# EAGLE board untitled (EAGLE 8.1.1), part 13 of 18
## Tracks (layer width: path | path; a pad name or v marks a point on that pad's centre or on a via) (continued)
S$13047 (continued)
  Bottom 0: 298.18,114.21 298.3,114.24
S$13048
  Bottom 0: 298.3,114.24 297.54,113.48
S$13049
  Bottom 0: 297.54,113.48 297.49,113.43
S$13050
  Bottom 0: 297.49,113.43 297.45,113.37
S$13051
  Bottom 0: 297.45,113.37 297.42,113.3
S$13052
  Bottom 0: 297.42,113.3 297.41,113.24
S$13053
  Bottom 0: 297.41,113.24 297.4,113.17
S$13054
  Bottom 0: 297.4,113.17 297.4,112
S$13055
  Bottom 0: 297.4,112 296.57,111.17
S$13056
  Bottom 0: 248.77,112.57 248.77,125.97
S$13057
  Bottom 0: 248.77,125.97 248.84,126.02
S$13058
  Bottom 0: 248.84,126.02 248.97,126.23
S$13059
  Bottom 0: 248.97,126.23 249.02,126.48
S$13060
  Bottom 0: 249.02,126.48 248.97,126.73
S$13061
  Bottom 0: 248.97,126.73 248.84,126.94
S$13062
  Bottom 0: 248.84,126.94 248.77,127
S$13063
  Bottom 0: 248.77,127 248.77,135.59
S$13064
  Bottom 0: 248.77,135.59 257.07,143.89
S$13065
  Bottom 0: 257.07,143.89 257.07,143.68
S$13066
  Bottom 0: 257.07,143.68 257.15,143.37
S$13067
  Bottom 0: 257.15,143.37 257.32,143.09
S$13068
  Bottom 0: 257.32,143.09 257.56,142.87
S$13069
  Bottom 0: 257.56,142.87 257.85,142.72
S$13070
  Bottom 0: 257.85,142.72 258.17,142.66
S$13071
  Bottom 0: 258.17,142.66 258.5,142.68
S$13072
  Bottom 0: 258.5,142.68 258.71,142.75
S$13073
  Bottom 0: 258.71,142.75 259.77,141.7
S$13074
  Bottom 0: 259.77,141.7 259.73,141.68
S$13075
  Bottom 0: 259.73,141.68 259.67,141.62
S$13076
  Bottom 0: 259.67,141.62 259.63,141.55
S$13077
  Bottom 0: 259.63,141.55 259.62,141.48
S$13078
  Bottom 0: 259.62,141.48 259.62,139.7
S$13079
  Bottom 0: 259.62,139.7 259.63,139.62
S$13080
  Bottom 0: 259.63,139.62 259.67,139.55
S$13081
  Bottom 0: 259.67,139.55 259.73,139.5
S$13082
  Bottom 0: 259.73,139.5 259.8,139.46
S$13083
  Bottom 0: 259.8,139.46 259.87,139.45
S$13084
  Bottom 0: 259.87,139.45 261.36,139.45
S$13085
  Bottom 0: 261.36,139.45 257.23,135.32
S$13086
  Bottom 0: 257.23,135.32 257.17,135.25
S$13087
  Bottom 0: 257.17,135.25 257.12,135.18
S$13088
  Bottom 0: 257.12,135.18 257.09,135.1
S$13089
  Bottom 0: 257.09,135.1 257.07,135.01
S$13090
  Bottom 0: 257.07,135.01 257.06,134.92
S$13091
  Bottom 0: 257.06,134.92 257.06,122.61
S$13092
  Bottom 0: 257.06,122.61 257.04,122.63
S$13093
  Bottom 0: 257.04,122.63 256.97,122.67
S$13094
  Bottom 0: 256.97,122.67 256.89,122.68
S$13095
  Bottom 0: 256.89,122.68 255.11,122.68
S$13096
  Bottom 0: 255.11,122.68 255.04,122.67
S$13097
  Bottom 0: 255.04,122.67 254.97,122.63
S$13098
  Bottom 0: 254.97,122.63 254.91,122.58
S$13099
  Bottom 0: 254.91,122.58 254.87,122.5
S$13100
  Bottom 0: 254.87,122.5 254.86,122.43
S$13101
  Bottom 0: 254.86,122.43 254.86,120.65
S$13102
  Bottom 0: 254.86,120.65 254.87,120.57
S$13103
  Bottom 0: 254.87,120.57 254.91,120.5
S$13104
  Bottom 0: 254.91,120.5 254.97,120.45
S$13105
  Bottom 0: 254.97,120.45 255.04,120.41
S$13106
  Bottom 0: 255.04,120.41 255.11,120.4
S$13107
  Bottom 0: 255.11,120.4 256.6,120.4
S$13108
  Bottom 0: 256.6,120.4 248.77,112.57
S$13109
  Bottom 0: 302.63,114.76 302.56,114.85
S$13110
  Bottom 0: 302.56,114.85 302.3,115.08
S$13111
  Bottom 0: 302.3,115.08 301.98,115.23
S$13112
  Bottom 0: 301.98,115.23 301.63,115.29
S$13113
  Bottom 0: 301.63,115.29 301.29,115.27
S$13114
  Bottom 0: 301.29,115.27 301.18,115.23
S$13115
  Bottom 0: 301.18,115.23 300.87,115.29
S$13116
  Bottom 0: 300.87,115.29 300.58,115.28
S$13117
  Bottom 0: 300.58,115.28 300.6,115.3
S$13118
  Bottom 0: 300.6,115.3 300.65,115.35
S$13119
  Bottom 0: 300.65,115.35 300.69,115.41
S$13120
  Bottom 0: 300.69,115.41 300.72,115.47
S$13121
  Bottom 0: 300.72,115.47 300.73,115.54
S$13122
  Bottom 0: 300.73,115.54 300.74,115.61
S$13123
  Bottom 0: 300.74,115.61 300.74,123.98
S$13124
  Bottom 0: 300.74,123.98 300.9,123.81
S$13125
  Bottom 0: 300.9,123.81 301.03,123.75
S$13126
  Bottom 0: 301.03,123.75 301.03,121.64
S$13127
  Bottom 0: 301.03,121.64 301.03,121.54
S$13128
  Bottom 0: 301.03,121.54 301.05,121.46
S$13129
  Bottom 0: 301.05,121.46 301.09,121.38
S$13130
  Bottom 0: 301.09,121.38 301.13,121.3
S$13131
  Bottom 0: 301.13,121.3 301.19,121.23
S$13132
  Bottom 0: 301.19,121.23 302.63,119.8
S$13133
  Bottom 0: 302.63,119.8 302.63,114.76
S$13134
  Bottom 0: 109.4,115.7 109.49,116.01
S$13135
  Bottom 0: 109.49,116.01 109.54,116.46
S$13136
  Bottom 0: 109.54,116.46 109.49,116.91
S$13137
  Bottom 0: 109.49,116.91 109.37,117.33
S$13138
  Bottom 0: 109.37,117.33 109.15,117.73
S$13139
  Bottom 0: 109.15,117.73 108.87,118.07
S$13140
  Bottom 0: 108.87,118.07 108.52,118.36
S$13141
  Bottom 0: 108.52,118.36 108.13,118.57
S$13142
  Bottom 0: 108.13,118.57 107.7,118.7
S$13143
  Bottom 0: 107.7,118.7 107.25,118.75
S$13144
  Bottom 0: 107.25,118.75 106.81,118.7
S$13145
  Bottom 0: 106.81,118.7 106.38,118.57
S$13146
  Bottom 0: 106.38,118.57 105.98,118.36
S$13147
  Bottom 0: 105.98,118.36 105.64,118.07
S$13148
  Bottom 0: 105.64,118.07 105.35,117.73
S$13149
  Bottom 0: 105.35,117.73 105.14,117.33
S$13150
  Bottom 0: 105.14,117.33 105.01,116.91
S$13151
  Bottom 0: 105.01,116.91 104.97,116.46
S$13152
  Bottom 0: 104.97,116.46 105.01,116.01
S$13153
  Bottom 0: 105.01,116.01 105.1,115.72
S$13154
  Bottom 0: 105.1,115.72 96.31,124.5
S$13155
  Bottom 0: 96.31,124.5 103.58,131.77
S$13156
  Bottom 0: 103.58,131.77 103.64,131.84
S$13157
  Bottom 0: 103.64,131.84 103.68,131.91
S$13158
  Bottom 0: 103.68,131.91 103.72,131.99
S$13159
  Bottom 0: 103.72,131.99 103.74,132.08
S$13160
  Bottom 0: 103.74,132.08 103.74,132.17
S$13161
  Bottom 0: 103.74,132.17 103.74,141.64
S$13162
  Bottom 0: 103.74,141.64 114.43,141.64
S$13163
  Bottom 0: 114.43,141.64 114.41,141.62
S$13164
  Bottom 0: 114.41,141.62 114.37,141.55
S$13165
  Bottom 0: 114.37,141.55 114.36,141.48
S$13166
  Bottom 0: 114.36,141.48 114.36,139.7
S$13167
  Bottom 0: 114.36,139.7 114.37,139.62
S$13168
  Bottom 0: 114.37,139.62 114.41,139.55
S$13169
  Bottom 0: 114.41,139.55 114.47,139.5
S$13170
  Bottom 0: 114.47,139.5 114.54,139.46
S$13171
  Bottom 0: 114.54,139.46 114.61,139.45
S$13172
  Bottom 0: 114.61,139.45 116.39,139.45
S$13173
  Bottom 0: 116.39,139.45 116.47,139.46
S$13174
  Bottom 0: 116.47,139.46 116.54,139.5
S$13175
  Bottom 0: 116.54,139.5 116.6,139.55
S$13176
  Bottom 0: 116.6,139.55 116.64,139.62
S$13177
  Bottom 0: 116.64,139.62 116.65,139.7
S$13178
  Bottom 0: 116.65,139.7 116.65,141.48
S$13179
  Bottom 0: 116.65,141.48 116.64,141.55
S$13180
  Bottom 0: 116.64,141.55 116.6,141.62
S$13181
  Bottom 0: 116.6,141.62 116.58,141.64
S$13182
  Bottom 0: 116.58,141.64 117.61,141.64
S$13183
  Bottom 0: 117.61,141.64 117.57,141.63
S$13184
  Bottom 0: 117.57,141.63 117.3,141.45
S$13185
  Bottom 0: 117.3,141.45 117.08,141.21
S$13186
  Bottom 0: 117.08,141.21 116.94,140.91
S$13187
  Bottom 0: 116.94,140.91 116.9,140.59
S$13188
  Bottom 0: 116.9,140.59 116.94,140.27
S$13189
  Bottom 0: 116.94,140.27 117.08,139.97
S$13190
  Bottom 0: 117.08,139.97 117.3,139.72
S$13191
  Bottom 0: 117.3,139.72 117.57,139.55
S$13192
  Bottom 0: 117.57,139.55 117.88,139.46
S$13193
  Bottom 0: 117.88,139.46 118.21,139.46
S$13194
  Bottom 0: 118.21,139.46 118.52,139.55
S$13195
  Bottom 0: 118.52,139.55 118.79,139.72
S$13196
  Bottom 0: 118.79,139.72 119,139.97
S$13197
  Bottom 0: 119,139.97 119.14,140.27
S$13198
  Bottom 0: 119.14,140.27 119.19,140.59
S$13199
  Bottom 0: 119.19,140.59 119.14,140.91
S$13200
  Bottom 0: 119.14,140.91 119,141.21
S$13201
  Bottom 0: 119,141.21 118.79,141.45
S$13202
  Bottom 0: 118.79,141.45 118.52,141.63
S$13203
  Bottom 0: 118.52,141.63 118.48,141.64
S$13204
  Bottom 0: 118.48,141.64 118.96,141.64
S$13205
  Bottom 0: 118.96,141.64 119.04,141.65
S$13206
  Bottom 0: 119.04,141.65 119.14,141.67
S$13207
  Bottom 0: 119.14,141.67 119.22,141.7
S$13208
  Bottom 0: 119.22,141.7 119.29,141.75
S$13209
  Bottom 0: 119.29,141.75 119.36,141.81
S$13210
  Bottom 0: 119.36,141.81 120.26,142.71
S$13211
  Bottom 0: 120.26,142.71 120.52,142.66
S$13212
  Bottom 0: 120.52,142.66 120.84,142.68
S$13213
  Bottom 0: 120.84,142.68 121.15,142.78
S$13214
  Bottom 0: 121.15,142.78 121.41,142.97
S$13215
  Bottom 0: 121.41,142.97 121.51,143.09
S$13216
  Bottom 0: 121.51,143.09 121.51,137.35
S$13217
  Bottom 0: 121.51,137.35 118.92,134.76
S$13218
  Bottom 0: 118.92,134.76 119.01,135.06
S$13219
  Bottom 0: 119.01,135.06 119.06,135.51
S$13220
  Bottom 0: 119.06,135.51 119.01,135.96
S$13221
  Bottom 0: 119.01,135.96 118.89,136.38
S$13222
  Bottom 0: 118.89,136.38 118.67,136.78
S$13223
  Bottom 0: 118.67,136.78 118.39,137.12
S$13224
  Bottom 0: 118.39,137.12 118.04,137.41
S$13225
  Bottom 0: 118.04,137.41 117.64,137.62
S$13226
  Bottom 0: 117.64,137.62 117.22,137.75
S$13227
  Bottom 0: 117.22,137.75 116.77,137.79
S$13228
  Bottom 0: 116.77,137.79 116.33,137.75
S$13229
  Bottom 0: 116.33,137.75 115.9,137.62
S$13230
  Bottom 0: 115.9,137.62 115.5,137.41
S$13231
  Bottom 0: 115.5,137.41 115.16,137.12
S$13232
  Bottom 0: 115.16,137.12 114.87,136.78
S$13233
  Bottom 0: 114.87,136.78 114.66,136.38
S$13234
  Bottom 0: 114.66,136.38 114.53,135.96
S$13235
  Bottom 0: 114.53,135.96 114.49,135.51
S$13236
  Bottom 0: 114.49,135.51 114.53,135.06
S$13237
  Bottom 0: 114.53,135.06 114.66,134.63
S$13238
  Bottom 0: 114.66,134.63 114.87,134.24
S$13239
  Bottom 0: 114.87,134.24 115.16,133.89
S$13240
  Bottom 0: 115.16,133.89 115.5,133.61
S$13241
  Bottom 0: 115.5,133.61 115.9,133.4
S$13242
  Bottom 0: 115.9,133.4 116.33,133.27
S$13243
  Bottom 0: 116.33,133.27 116.77,133.22
S$13244
  Bottom 0: 116.77,133.22 117.22,133.27
S$13245
  Bottom 0: 117.22,133.27 117.52,133.35
S$13246
  Bottom 0: 117.52,133.35 116.34,132.18
S$13247
  Bottom 0: 116.34,132.18 116.29,132.12
S$13248
  Bottom 0: 116.29,132.12 116.25,132.06
S$13249
  Bottom 0: 116.25,132.06 116.22,132
S$13250
  Bottom 0: 116.22,132 116.21,131.93
S$13251
  Bottom 0: 116.21,131.93 116.2,131.86
S$13252
  Bottom 0: 116.2,131.86 116.2,130.76
S$13253
  Bottom 0: 116.2,130.76 115.59,130.15
S$13254
  Bottom 0: 115.59,130.15 115.63,130.43
S$13255
  Bottom 0: 115.63,130.43 115.58,130.77
S$13256
  Bottom 0: 115.58,130.77 115.46,131.1
S$13257
  Bottom 0: 115.46,131.1 115.25,131.38
S$13258
  Bottom 0: 115.25,131.38 114.98,131.61
S$13259
  Bottom 0: 114.98,131.61 114.67,131.76
S$13260
  Bottom 0: 114.67,131.76 114.32,131.82
S$13261
  Bottom 0: 114.32,131.82 113.97,131.8
S$13262
  Bottom 0: 113.97,131.8 113.64,131.69
S$13263
  Bottom 0: 113.64,131.69 113.61,131.68
S$13264
  Bottom 0: 113.61,131.68 113.04,132.25
S$13265
  Bottom 0: 113.04,132.25 112.99,132.29
S$13266
  Bottom 0: 112.99,132.29 112.93,132.33
S$13267
  Bottom 0: 112.93,132.33 112.87,132.35
S$13268
  Bottom 0: 112.87,132.35 112.8,132.37
S$13269
  Bottom 0: 112.8,132.37 112.73,132.38
S$13270
  Bottom 0: 112.73,132.38 108.16,132.38
S$13271
  Bottom 0: 108.16,132.38 108.1,132.51
S$13272
  Bottom 0: 108.1,132.51 107.89,132.72
S$13273
  Bottom 0: 107.89,132.72 107.63,132.88
S$13274
  Bottom 0: 107.63,132.88 107.33,132.94
S$13275
  Bottom 0: 107.33,132.94 107.03,132.92
S$13276
  Bottom 0: 107.03,132.92 106.75,132.81
S$13277
  Bottom 0: 106.75,132.81 106.51,132.62
S$13278
  Bottom 0: 106.51,132.62 106.34,132.38
S$13279
  Bottom 0: 106.34,132.38 106.25,132.09
S$13280
  Bottom 0: 106.25,132.09 106.25,131.78
S$13281
  Bottom 0: 106.25,131.78 106.34,131.49
S$13282
  Bottom 0: 106.34,131.49 106.51,131.24
S$13283
  Bottom 0: 106.51,131.24 106.75,131.05
S$13284
  Bottom 0: 106.75,131.05 107.03,130.94
S$13285
  Bottom 0: 107.03,130.94 107.33,130.92
S$13286
  Bottom 0: 107.33,130.92 107.63,130.99
S$13287
  Bottom 0: 107.63,130.99 107.89,131.14
S$13288
  Bottom 0: 107.89,131.14 108.1,131.36
S$13289
  Bottom 0: 108.1,131.36 108.16,131.49
S$13290
  Bottom 0: 108.16,131.49 112.54,131.49
S$13291
  Bottom 0: 112.54,131.49 112.99,131.04
S$13292
  Bottom 0: 112.99,131.04 112.93,130.94
S$13293
  Bottom 0: 112.93,130.94 112.85,130.6
S$13294
  Bottom 0: 112.85,130.6 112.85,130.25
S$13295
  Bottom 0: 112.85,130.25 112.93,129.92
S$13296
  Bottom 0: 112.93,129.92 113.1,129.61
S$13297
  Bottom 0: 113.1,129.61 113.34,129.35
S$13298
  Bottom 0: 113.34,129.35 113.64,129.16
S$13299
  Bottom 0: 113.64,129.16 113.97,129.06
S$13300
  Bottom 0: 113.97,129.06 114.32,129.04
S$13301
  Bottom 0: 114.32,129.04 114.52,129.07
S$13302
  Bottom 0: 114.52,129.07 112.12,126.67
S$13303
  Bottom 0: 112.12,126.67 110.5,126.67
S$13304
  Bottom 0: 110.5,126.67 110.43,126.67
S$13305
  Bottom 0: 110.43,126.67 110.37,126.66
S$13306
  Bottom 0: 110.37,126.66 110.31,126.63
S$13307
  Bottom 0: 110.31,126.63 110.25,126.59
S$13308
  Bottom 0: 110.25,126.59 110.19,126.55
S$13309
  Bottom 0: 110.19,126.55 106.92,123.28
S$13310
  Bottom 0: 106.92,123.28 106.88,123.23
S$13311
  Bottom 0: 106.88,123.23 106.84,123.17
S$13312
  Bottom 0: 106.84,123.17 106.82,123.1
S$13313
  Bottom 0: 106.82,123.1 106.8,123.04
S$13314
  Bottom 0: 106.8,123.04 106.8,122.97
S$13315
  Bottom 0: 106.8,122.97 106.8,122.68
S$13316
  Bottom 0: 106.8,122.68 106.43,122.68
S$13317
  Bottom 0: 106.43,122.68 106.43,122.81
S$13318
  Bottom 0: 106.43,122.81 106.36,123.03
S$13319
  Bottom 0: 106.36,123.03 106.2,123.19
S$13320
  Bottom 0: 106.2,123.19 105.98,123.25
S$13321
  Bottom 0: 105.98,123.25 105.63,123.25
S$13322
  Bottom 0: 105.63,123.25 104.54,124.34
S$13323
  Bottom 0: 104.54,124.34 104.6,124.47
S$13324
  Bottom 0: 104.6,124.47 104.65,124.8
S$13325
  Bottom 0: 104.65,124.8 104.6,125.11
S$13326
  Bottom 0: 104.6,125.11 104.47,125.42
S$13327
  Bottom 0: 104.47,125.42 104.27,125.67
S$13328
  Bottom 0: 104.27,125.67 104,125.86
S$13329
  Bottom 0: 104,125.86 103.7,125.96
S$13330
  Bottom 0: 103.7,125.96 103.37,125.98
S$13331
  Bottom 0: 103.37,125.98 103.05,125.92
S$13332
  Bottom 0: 103.05,125.92 102.76,125.77
S$13333
  Bottom 0: 102.76,125.77 102.53,125.55
S$13334
  Bottom 0: 102.53,125.55 102.36,125.27
S$13335
  Bottom 0: 102.36,125.27 102.27,124.96
S$13336
  Bottom 0: 102.27,124.96 102.27,124.63
S$13337
  Bottom 0: 102.27,124.63 102.36,124.32
S$13338
  Bottom 0: 102.36,124.32 102.53,124.04
S$13339
  Bottom 0: 102.53,124.04 102.76,123.82
S$13340
  Bottom 0: 102.76,123.82 103.05,123.67
S$13341
  Bottom 0: 103.05,123.67 103.37,123.61
S$13342
  Bottom 0: 103.37,123.61 103.7,123.63
S$13343
  Bottom 0: 103.7,123.63 103.92,123.7
S$13344
  Bottom 0: 103.92,123.7 104.97,122.65
S$13345
  Bottom 0: 104.97,122.65 104.94,122.63
S$13346
  Bottom 0: 104.94,122.63 104.89,122.58
S$13347
  Bottom 0: 104.89,122.58 104.85,122.5
S$13348
  Bottom 0: 104.85,122.5 104.84,122.43
S$13349
  Bottom 0: 104.84,122.43 104.84,120.65
S$13350
  Bottom 0: 104.84,120.65 104.85,120.57
S$13351
  Bottom 0: 104.85,120.57 104.89,120.5
S$13352
  Bottom 0: 104.89,120.5 104.94,120.45
S$13353
  Bottom 0: 104.94,120.45 105.02,120.41
S$13354
  Bottom 0: 105.02,120.41 105.09,120.4
S$13355
  Bottom 0: 105.09,120.4 106.61,120.4
S$13356
  Bottom 0: 106.61,120.4 104.36,118.15
S$13357
  Bottom 0: 104.36,118.15 104.12,118.12
S$13358
  Bottom 0: 104.12,118.12 103.9,118.01
S$13359
  Bottom 0: 103.9,118.01 103.73,117.83
S$13360
  Bottom 0: 103.73,117.83 103.64,117.59
S$13361
  Bottom 0: 103.64,117.59 103.64,117.34
S$13362
  Bottom 0: 103.64,117.34 103.73,117.1
S$13363
  Bottom 0: 103.73,117.1 103.9,116.92
S$13364
  Bottom 0: 103.9,116.92 104.12,116.8
S$13365
  Bottom 0: 104.12,116.8 104.37,116.78
S$13366
  Bottom 0: 104.37,116.78 104.62,116.85
S$13367
  Bottom 0: 104.62,116.85 104.82,117
S$13368
  Bottom 0: 104.82,117 104.95,117.22
S$13369
  Bottom 0: 104.95,117.22 105,117.47
S$13370
  Bottom 0: 105,117.47 104.99,117.51
S$13371
  Bottom 0: 104.99,117.51 107.55,120.08
S$13372
  Bottom 0: 107.55,120.08 107.59,120.13
S$13373
  Bottom 0: 107.59,120.13 107.64,120.19
S$13374
  Bottom 0: 107.64,120.19 107.66,120.25
S$13375
  Bottom 0: 107.66,120.25 107.67,120.32
S$13376
  Bottom 0: 107.67,120.32 107.68,120.39
S$13377
  Bottom 0: 107.68,120.39 107.68,120.79
S$13378
  Bottom 0: 107.68,120.79 107.78,120.67
S$13379
  Bottom 0: 107.78,120.67 108.05,120.5
S$13380
  Bottom 0: 108.05,120.5 108.36,120.41
S$13381
  Bottom 0: 108.36,120.41 108.69,120.41
S$13382
  Bottom 0: 108.69,120.41 109,120.5
S$13383
  Bottom 0: 109,120.5 109.27,120.67
S$13384
  Bottom 0: 109.27,120.67 109.48,120.92
S$13385
  Bottom 0: 109.48,120.92 109.62,121.22
S$13386
  Bottom 0: 109.62,121.22 109.67,121.54
S$13387
  Bottom 0: 109.67,121.54 109.62,121.86
S$13388
  Bottom 0: 109.62,121.86 109.48,122.16
S$13389
  Bottom 0: 109.48,122.16 109.27,122.4
S$13390
  Bottom 0: 109.27,122.4 109,122.58
S$13391
  Bottom 0: 109,122.58 108.69,122.67
S$13392
  Bottom 0: 108.69,122.67 108.36,122.67
S$13393
  Bottom 0: 108.36,122.67 108.05,122.58
S$13394
  Bottom 0: 108.05,122.58 107.78,122.4
S$13395
  Bottom 0: 107.78,122.4 107.68,122.29
S$13396
  Bottom 0: 107.68,122.29 107.68,122.78
S$13397
  Bottom 0: 107.68,122.78 109.9,125
S$13398
  Bottom 0: 109.9,125 109.89,124.96
S$13399
  Bottom 0: 109.89,124.96 109.89,124.63
S$13400
  Bottom 0: 109.89,124.63 109.98,124.32
S$13401
  Bottom 0: 109.98,124.32 110.15,124.04
S$13402
  Bottom 0: 110.15,124.04 110.38,123.82
S$13403
  Bottom 0: 110.38,123.82 110.5,123.76
S$13404
  Bottom 0: 110.5,123.76 110.5,116.8
S$13405
  Bottom 0: 110.5,116.8 109.4,115.7
S$13406
  Bottom 0: 107.33,138.54 107.63,138.61
S$13407
  Bottom 0: 107.63,138.61 107.89,138.76
S$13408
  Bottom 0: 107.89,138.76 108.1,138.98
S$13409
  Bottom 0: 108.1,138.98 108.23,139.25
S$13410
  Bottom 0: 108.23,139.25 108.28,139.55
S$13411
  Bottom 0: 108.28,139.55 108.23,139.85
S$13412
  Bottom 0: 108.23,139.85 108.1,140.13
S$13413
  Bottom 0: 108.1,140.13 107.89,140.34
S$13414
  Bottom 0: 107.89,140.34 107.63,140.5
S$13415
  Bottom 0: 107.63,140.5 107.33,140.56
S$13416
  Bottom 0: 107.33,140.56 107.03,140.54
S$13417
  Bottom 0: 107.03,140.54 106.75,140.43
S$13418
  Bottom 0: 106.75,140.43 106.51,140.24
S$13419
  Bottom 0: 106.51,140.24 106.34,140
S$13420
  Bottom 0: 106.34,140 106.25,139.71
S$13421
  Bottom 0: 106.25,139.71 106.25,139.4
S$13422
  Bottom 0: 106.25,139.4 106.34,139.11
S$13423
  Bottom 0: 106.34,139.11 106.51,138.86
S$13424
  Bottom 0: 106.51,138.86 106.75,138.67
S$13425
  Bottom 0: 106.75,138.67 107.03,138.56
S$13426
  Bottom 0: 107.03,138.56 107.33,138.54
S$13427
  Bottom 0: 147.56,117.01 147.46,117.33
S$13428
  Bottom 0: 147.46,117.33 147.25,117.73
S$13429
  Bottom 0: 147.25,117.73 146.96,118.07
S$13430
  Bottom 0: 146.96,118.07 146.62,118.36
S$13431
  Bottom 0: 146.62,118.36 146.22,118.57
S$13432
  Bottom 0: 146.22,118.57 145.8,118.7
S$13433
  Bottom 0: 145.8,118.7 145.35,118.75
S$13434
  Bottom 0: 145.35,118.75 144.9,118.7
S$13435
  Bottom 0: 144.9,118.7 144.47,118.57
S$13436
  Bottom 0: 144.47,118.57 144.42,118.55
S$13437
  Bottom 0: 144.42,118.55 146.32,120.45
S$13438
  Bottom 0: 146.32,120.45 146.46,120.41
S$13439
  Bottom 0: 146.46,120.41 146.78,120.41
S$13440
  Bottom 0: 146.78,120.41 147.09,120.5
S$13441
  Bottom 0: 147.09,120.5 147.36,120.67
S$13442
  Bottom 0: 147.36,120.67 147.56,120.89
S$13443
  Bottom 0: 147.56,120.89 147.56,117.01
S$13444
  Bottom 0: 142.11,117.84 137.75,122.2
S$13445
  Bottom 0: 137.75,122.2 137.69,122.26
S$13446
  Bottom 0: 137.69,122.26 137.61,122.31
S$13447
  Bottom 0: 137.61,122.31 137.53,122.34
S$13448
  Bottom 0: 137.53,122.34 137.44,122.36
S$13449
  Bottom 0: 137.44,122.36 137.35,122.37
S$13450
  Bottom 0: 137.35,122.37 128.34,122.37
S$13451
  Bottom 0: 128.34,122.37 128.31,122.4
S$13452
  Bottom 0: 128.31,122.4 128.04,122.58
S$13453
  Bottom 0: 128.04,122.58 127.73,122.67
S$13454
  Bottom 0: 127.73,122.67 127.41,122.67
S$13455
  Bottom 0: 127.41,122.67 127.1,122.58
S$13456
  Bottom 0: 127.1,122.58 126.82,122.4
S$13457
  Bottom 0: 126.82,122.4 126.61,122.16
S$13458
  Bottom 0: 126.61,122.16 126.47,121.86
S$13459
  Bottom 0: 126.47,121.86 126.43,121.54
S$13460
  Bottom 0: 126.43,121.54 126.47,121.22
S$13461
  Bottom 0: 126.47,121.22 126.61,120.92
S$13462
  Bottom 0: 126.61,120.92 126.82,120.67
S$13463
  Bottom 0: 126.82,120.67 127,120.56
S$13464
  Bottom 0: 127,120.56 126.15,120.56
S$13465
  Bottom 0: 126.15,120.56 126.16,120.57
S$13466
  Bottom 0: 126.16,120.57 126.17,120.65
S$13467
  Bottom 0: 126.17,120.65 126.17,122.43
S$13468
  Bottom 0: 126.17,122.43 126.16,122.5
S$13469
  Bottom 0: 126.16,122.5 126.12,122.58
S$13470
  Bottom 0: 126.12,122.58 126.06,122.63
S$13471
  Bottom 0: 126.06,122.63 125.99,122.67
S$13472
  Bottom 0: 125.99,122.67 125.92,122.68
S$13473
  Bottom 0: 125.92,122.68 125.47,122.68
S$13474
  Bottom 0: 125.47,122.68 125.47,122.81
S$13475
  Bottom 0: 125.47,122.81 125.41,123.03
S$13476
  Bottom 0: 125.41,123.03 125.25,123.19
S$13477
  Bottom 0: 125.25,123.19 125.03,123.25
S$13478
  Bottom 0: 125.03,123.25 124.68,123.25
S$13479
  Bottom 0: 124.68,123.25 123.59,124.34
S$13480
  Bottom 0: 123.59,124.34 123.65,124.47
S$13481
  Bottom 0: 123.65,124.47 123.7,124.8
S$13482
  Bottom 0: 123.7,124.8 123.65,125.11
S$13483
  Bottom 0: 123.65,125.11 123.53,125.42
S$13484
  Bottom 0: 123.53,125.42 123.32,125.67
S$13485
  Bottom 0: 123.32,125.67 123.05,125.86
S$13486
  Bottom 0: 123.05,125.86 122.75,125.96
S$13487
  Bottom 0: 122.75,125.96 122.42,125.98
S$13488
  Bottom 0: 122.42,125.98 122.1,125.92
S$13489
  Bottom 0: 122.1,125.92 121.81,125.77
S$13490
  Bottom 0: 121.81,125.77 121.58,125.55
S$13491
  Bottom 0: 121.58,125.55 121.41,125.27
S$13492
  Bottom 0: 121.41,125.27 121.32,124.96
S$13493
  Bottom 0: 121.32,124.96 121.32,124.63
S$13494
  Bottom 0: 121.32,124.63 121.41,124.32
S$13495
  Bottom 0: 121.41,124.32 121.58,124.04
S$13496
  Bottom 0: 121.58,124.04 121.81,123.82
S$13497
  Bottom 0: 121.81,123.82 122.1,123.67
S$13498
  Bottom 0: 122.1,123.67 122.42,123.61
S$13499
  Bottom 0: 122.42,123.61 122.75,123.63
S$13500
  Bottom 0: 122.75,123.63 122.97,123.7
S$13501
  Bottom 0: 122.97,123.7 124.02,122.65
S$13502
  Bottom 0: 124.02,122.65 123.99,122.63
S$13503
  Bottom 0: 123.99,122.63 123.94,122.58
S$13504
  Bottom 0: 123.94,122.58 123.9,122.5
S$13505
  Bottom 0: 123.9,122.5 123.89,122.43
S$13506
  Bottom 0: 123.89,122.43 123.89,120.65
S$13507
  Bottom 0: 123.89,120.65 123.9,120.57
S$13508
  Bottom 0: 123.9,120.57 123.91,120.56
S$13509
  Bottom 0: 123.91,120.56 117.79,120.56
S$13510
  Bottom 0: 117.79,120.56 117.75,120.8
S$13511
  Bottom 0: 117.75,120.8 117.62,121.08
S$13512
  Bottom 0: 117.62,121.08 117.42,121.3
S$13513
  Bottom 0: 117.42,121.3 117.16,121.45
S$13514
  Bottom 0: 117.16,121.45 116.86,121.51
S$13515
  Bottom 0: 116.86,121.51 116.81,121.51
S$13516
  Bottom 0: 116.81,121.51 123.67,128.37
S$13517
  Bottom 0: 123.67,128.37 137.68,128.37
S$13518
  Bottom 0: 137.68,128.37 137.75,128.38
S$13519
  Bottom 0: 137.75,128.38 137.81,128.39
S$13520
  Bottom 0: 137.81,128.39 137.88,128.42
S$13521
  Bottom 0: 137.88,128.42 137.94,128.46
S$13522
  Bottom 0: 137.94,128.46 137.99,128.5
S$13523
  Bottom 0: 137.99,128.5 149.31,139.82
S$13524
  Bottom 0: 149.31,139.82 149.33,139.84
S$13525
  Bottom 0: 149.33,139.84 149.33,138.24
S$13526
  Bottom 0: 149.33,138.24 143.87,132.78
S$13527
  Bottom 0: 143.87,132.78 143.82,132.72
S$13528
  Bottom 0: 143.82,132.72 143.78,132.66
S$13529
  Bottom 0: 143.78,132.66 143.76,132.6
S$13530
  Bottom 0: 143.76,132.6 143.74,132.53
S$13531
  Bottom 0: 143.74,132.53 143.74,132.46
S$13532
  Bottom 0: 143.74,132.46 143.74,128.37
S$13533
  Bottom 0: 143.74,128.37 143.74,128.3
S$13534
  Bottom 0: 143.74,128.3 143.76,128.23
S$13535
  Bottom 0: 143.76,128.23 143.78,128.17
S$13536
  Bottom 0: 143.78,128.17 143.82,128.11
S$13537
  Bottom 0: 143.82,128.11 143.87,128.06
S$13538
  Bottom 0: 143.87,128.06 144.96,126.96
S$13539
  Bottom 0: 144.96,126.96 144.96,126.79
S$13540
  Bottom 0: 144.96,126.79 145.05,126.55
S$13541
  Bottom 0: 145.05,126.55 145.22,126.36
S$13542
  Bottom 0: 145.22,126.36 145.44,126.25
S$13543
  Bottom 0: 145.44,126.25 145.69,126.23
S$13544
  Bottom 0: 145.69,126.23 145.94,126.3
S$13545
  Bottom 0: 145.94,126.3 146.05,126.38
S$13546
  Bottom 0: 146.05,126.38 146.05,122.52
S$13547
  Bottom 0: 146.05,122.52 145.87,122.4
S$13548
  Bottom 0: 145.87,122.4 145.66,122.16
S$13549
  Bottom 0: 145.66,122.16 145.52,121.86
S$13550
  Bottom 0: 145.52,121.86 145.48,121.54
S$13551
  Bottom 0: 145.48,121.54 145.52,121.24
S$13552
  Bottom 0: 145.52,121.24 145.22,120.94
S$13553
  Bottom 0: 145.22,120.94 145.22,122.43
S$13554
  Bottom 0: 145.22,122.43 145.21,122.5
S$13555
  Bottom 0: 145.21,122.5 145.17,122.58
S$13556
  Bottom 0: 145.17,122.58 145.12,122.63
S$13557
  Bottom 0: 145.12,122.63 145.04,122.67
S$13558
  Bottom 0: 145.04,122.67 144.97,122.68
S$13559
  Bottom 0: 144.97,122.68 144.52,122.68
S$13560
  Bottom 0: 144.52,122.68 144.52,122.81
S$13561
  Bottom 0: 144.52,122.81 144.46,123.03
S$13562
  Bottom 0: 144.46,123.03 144.3,123.19
S$13563
  Bottom 0: 144.3,123.19 144.08,123.25
S$13564
  Bottom 0: 144.08,123.25 143.72,123.25
S$13565
  Bottom 0: 143.72,123.25 142.64,124.33
S$13566
  Bottom 0: 142.64,124.33 142.7,124.47
S$13567
  Bottom 0: 142.7,124.47 142.75,124.79
S$13568
  Bottom 0: 142.75,124.79 142.7,125.11
S$13569
  Bottom 0: 142.7,125.11 142.57,125.41
S$13570
  Bottom 0: 142.57,125.41 142.37,125.66
S$13571
  Bottom 0: 142.37,125.66 142.1,125.85
S$13572
  Bottom 0: 142.1,125.85 141.8,125.96
S$13573
  Bottom 0: 141.8,125.96 141.47,125.98
S$13574
  Bottom 0: 141.47,125.98 141.15,125.91
S$13575
  Bottom 0: 141.15,125.91 140.86,125.77
S$13576
  Bottom 0: 140.86,125.77 140.63,125.54
S$13577
  Bottom 0: 140.63,125.54 140.46,125.27
S$13578
  Bottom 0: 140.46,125.27 140.37,124.95
S$13579
  Bottom 0: 140.37,124.95 140.37,124.63
S$13580
  Bottom 0: 140.37,124.63 140.46,124.31
S$13581
  Bottom 0: 140.46,124.31 140.63,124.04
S$13582
  Bottom 0: 140.63,124.04 140.86,123.81
S$13583
  Bottom 0: 140.86,123.81 141.15,123.67
S$13584
  Bottom 0: 141.15,123.67 141.47,123.6
S$13585
  Bottom 0: 141.47,123.6 141.8,123.62
S$13586
  Bottom 0: 141.8,123.62 142.02,123.7
S$13587
  Bottom 0: 142.02,123.7 143.07,122.65
S$13588
  Bottom 0: 143.07,122.65 143.04,122.63
S$13589
  Bottom 0: 143.04,122.63 142.99,122.58
S$13590
  Bottom 0: 142.99,122.58 142.95,122.5
S$13591
  Bottom 0: 142.95,122.5 142.94,122.43
S$13592
  Bottom 0: 142.94,122.43 142.94,120.65
S$13593
  Bottom 0: 142.94,120.65 142.95,120.57
S$13594
  Bottom 0: 142.95,120.57 142.99,120.5
S$13595
  Bottom 0: 142.99,120.5 143.04,120.45
S$13596
  Bottom 0: 143.04,120.45 143.11,120.41
S$13597
  Bottom 0: 143.11,120.41 143.19,120.4
S$13598
  Bottom 0: 143.19,120.4 144.67,120.4
S$13599
  Bottom 0: 144.67,120.4 142.11,117.84
S$13600
  Bottom 0: 130.04,123.61 130.37,123.63
S$13601
  Bottom 0: 130.37,123.63 130.67,123.73
S$13602
  Bottom 0: 130.67,123.73 130.94,123.92
S$13603
  Bottom 0: 130.94,123.92 131.15,124.18
S$13604
  Bottom 0: 131.15,124.18 131.27,124.47
S$13605
  Bottom 0: 131.27,124.47 131.32,124.8
S$13606
  Bottom 0: 131.32,124.8 131.27,125.11
S$13607
  Bottom 0: 131.27,125.11 131.15,125.42
S$13608
  Bottom 0: 131.15,125.42 130.94,125.67
S$13609
  Bottom 0: 130.94,125.67 130.67,125.86
S$13610
  Bottom 0: 130.67,125.86 130.37,125.96
S$13611
  Bottom 0: 130.37,125.96 130.04,125.98
S$13612
  Bottom 0: 130.04,125.98 129.72,125.92
S$13613
  Bottom 0: 129.72,125.92 129.43,125.77
S$13614
  Bottom 0: 129.43,125.77 129.2,125.55
S$13615
  Bottom 0: 129.2,125.55 129.03,125.27
S$13616
  Bottom 0: 129.03,125.27 128.94,124.96
S$13617
  Bottom 0: 128.94,124.96 128.94,124.63
S$13618
  Bottom 0: 128.94,124.63 129.03,124.32
S$13619
  Bottom 0: 129.03,124.32 129.2,124.04
S$13620
  Bottom 0: 129.2,124.04 129.43,123.82
S$13621
  Bottom 0: 129.43,123.82 129.72,123.67
S$13622
  Bottom 0: 129.72,123.67 130.04,123.61
S$13623
  Bottom 0: 90.08,120.59 90.21,120.67
S$13624
  Bottom 0: 90.21,120.67 90.43,120.92
S$13625
  Bottom 0: 90.43,120.92 90.56,121.22
S$13626
  Bottom 0: 90.56,121.22 90.61,121.54
S$13627
  Bottom 0: 90.61,121.54 90.56,121.86
S$13628
  Bottom 0: 90.56,121.86 90.43,122.16
S$13629
  Bottom 0: 90.43,122.16 90.21,122.4
S$13630
  Bottom 0: 90.21,122.4 90.04,122.52
S$13631
  Bottom 0: 90.04,122.52 90.04,131.01
S$13632
  Bottom 0: 90.04,131.01 91.23,132.2
S$13633
  Bottom 0: 91.23,132.2 91.26,132.2
S$13634
  Bottom 0: 91.26,132.2 91.34,132.22
S$13635
  Bottom 0: 91.34,132.22 91.42,132.25
S$13636
  Bottom 0: 91.42,132.25 91.5,132.3
S$13637
  Bottom 0: 91.5,132.3 91.57,132.36
S$13638
  Bottom 0: 91.57,132.36 95.64,136.43
S$13639
  Bottom 0: 95.64,136.43 95.61,136.38
S$13640
  Bottom 0: 95.61,136.38 95.48,135.96
S$13641
  Bottom 0: 95.48,135.96 95.44,135.51
S$13642
  Bottom 0: 95.44,135.51 95.48,135.06
S$13643
  Bottom 0: 95.48,135.06 95.61,134.63
S$13644
  Bottom 0: 95.61,134.63 95.82,134.24
S$13645
  Bottom 0: 95.82,134.24 96.11,133.89
S$13646
  Bottom 0: 96.11,133.89 96.45,133.61
S$13647
  Bottom 0: 96.45,133.61 96.85,133.4
S$13648
  Bottom 0: 96.85,133.4 97.28,133.27
S$13649
  Bottom 0: 97.28,133.27 97.72,133.22
S$13650
  Bottom 0: 97.72,133.22 98.17,133.27
S$13651
  Bottom 0: 98.17,133.27 98.59,133.4
S$13652
  Bottom 0: 98.59,133.4 98.99,133.61
S$13653
  Bottom 0: 98.99,133.61 99.34,133.89
S$13654
  Bottom 0: 99.34,133.89 99.62,134.24
S$13655
  Bottom 0: 99.62,134.24 99.83,134.63
S$13656
  Bottom 0: 99.83,134.63 99.96,135.06
S$13657
  Bottom 0: 99.96,135.06 100.01,135.51
S$13658
  Bottom 0: 100.01,135.51 99.96,135.96
S$13659
  Bottom 0: 99.96,135.96 99.83,136.38
S$13660
  Bottom 0: 99.83,136.38 99.62,136.78
S$13661
  Bottom 0: 99.62,136.78 99.34,137.12
S$13662
  Bottom 0: 99.34,137.12 98.99,137.41
S$13663
  Bottom 0: 98.99,137.41 98.59,137.62
S$13664
  Bottom 0: 98.59,137.62 98.17,137.75
S$13665
  Bottom 0: 98.17,137.75 97.72,137.79
S$13666
  Bottom 0: 97.72,137.79 97.28,137.75
S$13667
  Bottom 0: 97.28,137.75 96.85,137.62
S$13668
  Bottom 0: 96.85,137.62 96.8,137.6
S$13669
  Bottom 0: 96.8,137.6 98.7,139.5
S$13670
  Bottom 0: 98.7,139.5 98.83,139.46
S$13671
  Bottom 0: 98.83,139.46 99.16,139.46
S$13672
  Bottom 0: 99.16,139.46 99.47,139.55
S$13673
  Bottom 0: 99.47,139.55 99.74,139.72
S$13674
  Bottom 0: 99.74,139.72 99.95,139.97
S$13675
  Bottom 0: 99.95,139.97 100.09,140.27
S$13676
  Bottom 0: 100.09,140.27 100.14,140.59
S$13677
  Bottom 0: 100.14,140.59 100.14,140.61
S$13678
  Bottom 0: 100.14,140.61 101.09,139.65
S$13679
  Bottom 0: 101.09,139.65 101.09,134.28
S$13680
  Bottom 0: 101.09,134.28 100.94,134.23
S$13681
  Bottom 0: 100.94,134.23 100.64,134.05
S$13682
  Bottom 0: 100.64,134.05 100.4,133.79
S$13683
  Bottom 0: 100.4,133.79 100.23,133.48
S$13684
  Bottom 0: 100.23,133.48 100.15,133.14
S$13685
  Bottom 0: 100.15,133.14 100.15,132.79
S$13686
  Bottom 0: 100.15,132.79 100.23,132.46
S$13687
  Bottom 0: 100.23,132.46 100.4,132.15
S$13688
  Bottom 0: 100.4,132.15 100.64,131.89
S$13689
  Bottom 0: 100.64,131.89 100.94,131.7
S$13690
  Bottom 0: 100.94,131.7 101.27,131.6
S$13691
  Bottom 0: 101.27,131.6 101.62,131.58
S$13692
  Bottom 0: 101.62,131.58 101.81,131.61
S$13693
  Bottom 0: 101.81,131.61 95.49,125.29
S$13694
  Bottom 0: 95.49,125.29 95.48,125.3
S$13695
  Bottom 0: 95.48,125.3 95.4,125.33
S$13696
  Bottom 0: 95.4,125.33 95.31,125.35
S$13697
  Bottom 0: 95.31,125.35 95.22,125.36
S$13698
  Bottom 0: 95.22,125.36 93.06,125.36
S$13699
  Bottom 0: 93.06,125.36 93.04,125.41
S$13700
  Bottom 0: 93.04,125.41 92.83,125.66
S$13701
  Bottom 0: 92.83,125.66 92.57,125.85
S$13702
  Bottom 0: 92.57,125.85 92.26,125.96
S$13703
  Bottom 0: 92.26,125.96 91.94,125.98
S$13704
  Bottom 0: 91.94,125.98 91.62,125.91
S$13705
  Bottom 0: 91.62,125.91 91.33,125.77
S$13706
  Bottom 0: 91.33,125.77 91.09,125.54
S$13707
  Bottom 0: 91.09,125.54 90.92,125.27
S$13708
  Bottom 0: 90.92,125.27 90.83,124.95
S$13709
  Bottom 0: 90.83,124.95 90.83,124.63
S$13710
  Bottom 0: 90.83,124.63 90.92,124.31
S$13711
  Bottom 0: 90.92,124.31 91.09,124.04
S$13712
  Bottom 0: 91.09,124.04 91.33,123.81
S$13713
  Bottom 0: 91.33,123.81 91.62,123.67
S$13714
  Bottom 0: 91.62,123.67 91.94,123.6
S$13715
  Bottom 0: 91.94,123.6 92.26,123.62
S$13716
  Bottom 0: 92.26,123.62 92.57,123.73
S$13717
  Bottom 0: 92.57,123.73 92.83,123.92
S$13718
  Bottom 0: 92.83,123.92 93.04,124.17
S$13719
  Bottom 0: 93.04,124.17 93.06,124.22
S$13720
  Bottom 0: 93.06,124.22 94.99,124.22
S$13721
  Bottom 0: 94.99,124.22 95.11,124.1
S$13722
  Bottom 0: 95.11,124.1 97.7,121.51
S$13723
  Bottom 0: 97.7,121.51 97.51,121.49
S$13724
  Bottom 0: 97.51,121.49 97.23,121.38
S$13725
  Bottom 0: 97.23,121.38 96.99,121.19
S$13726
  Bottom 0: 96.99,121.19 96.82,120.94
S$13727
  Bottom 0: 96.82,120.94 96.73,120.66
S$13728
  Bottom 0: 96.73,120.66 96.73,120.59
S$13729
  Bottom 0: 96.73,120.59 90.08,120.59
S$13730
  Bottom 0: 95.27,129.04 95.62,129.1
S$13731
  Bottom 0: 95.62,129.1 95.93,129.25
S$13732
  Bottom 0: 95.93,129.25 96.2,129.47
S$13733
  Bottom 0: 96.2,129.47 96.41,129.76
S$13734
  Bottom 0: 96.41,129.76 96.53,130.08
S$13735
  Bottom 0: 96.53,130.08 96.58,130.43
S$13736
  Bottom 0: 96.58,130.43 96.53,130.77
S$13737
  Bottom 0: 96.53,130.77 96.41,131.1
S$13738
  Bottom 0: 96.41,131.1 96.2,131.38
S$13739
  Bottom 0: 96.2,131.38 95.93,131.61
S$13740
  Bottom 0: 95.93,131.61 95.62,131.76
S$13741
  Bottom 0: 95.62,131.76 95.27,131.82
S$13742
  Bottom 0: 95.27,131.82 94.92,131.8
S$13743
  Bottom 0: 94.92,131.8 94.59,131.69
S$13744
  Bottom 0: 94.59,131.69 94.3,131.51
S$13745
  Bottom 0: 94.3,131.51 94.05,131.25
S$13746
  Bottom 0: 94.05,131.25 93.88,130.94
S$13747
  Bottom 0: 93.88,130.94 93.8,130.6
S$13748
  Bottom 0: 93.8,130.6 93.8,130.25
S$13749
  Bottom 0: 93.8,130.25 93.88,129.92
S$13750
  Bottom 0: 93.88,129.92 94.05,129.61
S$13751
  Bottom 0: 94.05,129.61 94.3,129.35
S$13752
  Bottom 0: 94.3,129.35 94.59,129.16
S$13753
  Bottom 0: 94.59,129.16 94.92,129.06
S$13754
  Bottom 0: 94.92,129.06 95.27,129.04
S$13755
  Bottom 0: 185.7,122.11 185.68,122.16
S$13756
  Bottom 0: 185.68,122.16 185.47,122.4
S$13757
  Bottom 0: 185.47,122.4 185.19,122.58
S$13758
  Bottom 0: 185.19,122.58 185.16,122.59
S$13759
  Bottom 0: 185.16,122.59 185.64,122.59
S$13760
  Bottom 0: 185.64,122.59 185.72,122.6
S$13761
  Bottom 0: 185.72,122.6 185.82,122.62
S$13762
  Bottom 0: 185.82,122.62 185.9,122.65
S$13763
  Bottom 0: 185.9,122.65 185.97,122.7
S$13764
  Bottom 0: 185.97,122.7 186.04,122.76
S$13765
  Bottom 0: 186.04,122.76 186.94,123.66
S$13766
  Bottom 0: 186.94,123.66 187.2,123.61
S$13767
  Bottom 0: 187.2,123.61 187.52,123.63
S$13768
  Bottom 0: 187.52,123.63 187.83,123.73
S$13769
  Bottom 0: 187.83,123.73 188.09,123.92
S$13770
  Bottom 0: 188.09,123.92 188.3,124.18
S$13771
  Bottom 0: 188.3,124.18 188.43,124.47
S$13772
  Bottom 0: 188.43,124.47 188.47,124.8
S$13773
  Bottom 0: 188.47,124.8 188.43,125.11
S$13774
  Bottom 0: 188.43,125.11 188.3,125.42
S$13775
  Bottom 0: 188.3,125.42 188.09,125.67
S$13776
  Bottom 0: 188.09,125.67 187.83,125.86
S$13777
  Bottom 0: 187.83,125.86 187.52,125.96
S$13778
  Bottom 0: 187.52,125.96 187.2,125.98
S$13779
  Bottom 0: 187.2,125.98 186.88,125.92
S$13780
  Bottom 0: 186.88,125.92 186.59,125.77
S$13781
  Bottom 0: 186.59,125.77 186.35,125.55
S$13782
  Bottom 0: 186.35,125.55 186.18,125.27
S$13783
  Bottom 0: 186.18,125.27 186.1,124.96
S$13784
  Bottom 0: 186.1,124.96 186.1,124.63
S$13785
  Bottom 0: 186.1,124.63 186.14,124.47
S$13786
  Bottom 0: 186.14,124.47 185.41,123.73
S$13787
  Bottom 0: 185.41,123.73 180.19,123.73
S$13788
  Bottom 0: 180.19,123.73 180.21,123.73
S$13789
  Bottom 0: 180.21,123.73 180.47,123.92
S$13790
  Bottom 0: 180.47,123.92 180.68,124.18
S$13791
  Bottom 0: 180.68,124.18 180.81,124.47
S$13792
  Bottom 0: 180.81,124.47 180.85,124.8
S$13793
  Bottom 0: 180.85,124.8 180.81,125.11
S$13794
  Bottom 0: 180.81,125.11 180.68,125.42
S$13795
  Bottom 0: 180.68,125.42 180.47,125.67
S$13796
  Bottom 0: 180.47,125.67 180.21,125.86
S$13797
  Bottom 0: 180.21,125.86 179.9,125.96
S$13798
  Bottom 0: 179.9,125.96 179.58,125.98
S$13799
  Bottom 0: 179.58,125.98 179.26,125.92
S$13800
  Bottom 0: 179.26,125.92 178.97,125.77
S$13801
  Bottom 0: 178.97,125.77 178.74,125.55
S$13802
  Bottom 0: 178.74,125.55 178.66,125.42
S$13803
  Bottom 0: 178.66,125.42 178.66,126.22
S$13804
  Bottom 0: 178.66,126.22 179.79,127.35
S$13805
  Bottom 0: 179.79,127.35 179.85,127.42
S$13806
  Bottom 0: 179.85,127.42 179.9,127.49
S$13807
  Bottom 0: 179.9,127.49 179.93,127.57
S$13808
  Bottom 0: 179.93,127.57 179.95,127.66
S$13809
  Bottom 0: 179.95,127.66 179.96,127.75
S$13810
  Bottom 0: 179.96,127.75 179.96,141.64
S$13811
  Bottom 0: 179.96,141.64 188.25,141.64
S$13812
  Bottom 0: 188.25,141.64 188.2,141.58
S$13813
  Bottom 0: 188.2,141.58 188.11,141.35
S$13814
  Bottom 0: 188.11,141.35 188.11,141.09
S$13815
  Bottom 0: 188.11,141.09 188.2,140.86
S$13816
  Bottom 0: 188.2,140.86 188.37,140.67
S$13817
  Bottom 0: 188.37,140.67 188.59,140.56
S$13818
  Bottom 0: 188.59,140.56 190.8,138.35
S$13819
  Bottom 0: 190.8,138.35 190.85,138.31
S$13820
  Bottom 0: 190.85,138.31 190.91,138.27
S$13821
  Bottom 0: 190.91,138.27 190.97,138.25
S$13822
  Bottom 0: 190.97,138.25 191.04,138.23
S$13823
  Bottom 0: 191.04,138.23 191.11,138.23
S$13824
  Bottom 0: 191.11,138.23 193.03,138.23
S$13825
  Bottom 0: 193.03,138.23 193.54,137.71
S$13826
  Bottom 0: 193.54,137.71 193.42,137.75
S$13827
  Bottom 0: 193.42,137.75 192.97,137.79
S$13828
  Bottom 0: 192.97,137.79 192.53,137.75
S$13829
  Bottom 0: 192.53,137.75 192.1,137.62
S$13830
  Bottom 0: 192.1,137.62 191.7,137.41
S$13831
  Bottom 0: 191.7,137.41 191.36,137.12
S$13832
  Bottom 0: 191.36,137.12 191.07,136.78
S$13833
  Bottom 0: 191.07,136.78 190.86,136.38
S$13834
  Bottom 0: 190.86,136.38 190.73,135.96
S$13835
  Bottom 0: 190.73,135.96 190.69,135.51
S$13836
  Bottom 0: 190.69,135.51 190.73,135.06
S$13837
  Bottom 0: 190.73,135.06 190.86,134.63
S$13838
  Bottom 0: 190.86,134.63 191.07,134.24
S$13839
  Bottom 0: 191.07,134.24 191.36,133.89
S$13840
  Bottom 0: 191.36,133.89 191.7,133.61
S$13841
  Bottom 0: 191.7,133.61 192.1,133.4
S$13842
  Bottom 0: 192.1,133.4 192.53,133.27
S$13843
  Bottom 0: 192.53,133.27 192.97,133.22
S$13844
  Bottom 0: 192.97,133.22 193.42,133.27
S$13845
  Bottom 0: 193.42,133.27 193.85,133.4
S$13846
  Bottom 0: 193.85,133.4 194.24,133.61
S$13847
  Bottom 0: 194.24,133.61 194.59,133.89
S$13848
  Bottom 0: 194.59,133.89 194.87,134.24
S$13849
  Bottom 0: 194.87,134.24 195.09,134.63
S$13850
  Bottom 0: 195.09,134.63 195.21,135.06
S$13851
  Bottom 0: 195.21,135.06 195.26,135.51
S$13852
  Bottom 0: 195.26,135.51 195.21,135.96
S$13853
  Bottom 0: 195.21,135.96 195.18,136.07
S$13854
  Bottom 0: 195.18,136.07 196.34,134.91
S$13855
  Bottom 0: 196.34,134.91 196.34,134.28
S$13856
  Bottom 0: 196.34,134.28 196.19,134.23
S$13857
  Bottom 0: 196.19,134.23 195.9,134.05
S$13858
  Bottom 0: 195.9,134.05 195.66,133.79
S$13859
  Bottom 0: 195.66,133.79 195.48,133.48
S$13860
  Bottom 0: 195.48,133.48 195.4,133.14
S$13861
  Bottom 0: 195.4,133.14 195.4,132.79
S$13862
  Bottom 0: 195.4,132.79 195.48,132.46
S$13863
  Bottom 0: 195.48,132.46 195.66,132.15
S$13864
  Bottom 0: 195.66,132.15 195.9,131.89
S$13865
  Bottom 0: 195.9,131.89 196.19,131.7
S$13866
  Bottom 0: 196.19,131.7 196.52,131.6
S$13867
  Bottom 0: 196.52,131.6 196.87,131.58
S$13868
  Bottom 0: 196.87,131.58 197.22,131.64
S$13869
  Bottom 0: 197.22,131.64 197.53,131.79
S$13870
  Bottom 0: 197.53,131.79 197.8,132.01
S$13871
  Bottom 0: 197.8,132.01 198.01,132.3
S$13872
  Bottom 0: 198.01,132.3 198.06,132.43
S$13873
  Bottom 0: 198.06,132.43 198.06,126.81
S$13874
  Bottom 0: 198.06,126.81 196.82,126.81
S$13875
  Bottom 0: 196.82,126.81 196.73,126.8
S$13876
  Bottom 0: 196.73,126.8 196.64,126.78
S$13877
  Bottom 0: 196.64,126.78 196.56,126.75
S$13878
  Bottom 0: 196.56,126.75 196.48,126.7
S$13879
  Bottom 0: 196.48,126.7 196.42,126.64
S$13880
  Bottom 0: 196.42,126.64 191.89,122.11
S$13881
  Bottom 0: 191.89,122.11 185.7,122.11
S$13882
  Bottom 0: 190.52,129.04 190.87,129.1
S$13883
  Bottom 0: 190.87,129.1 191.18,129.25
S$13884
  Bottom 0: 191.18,129.25 191.45,129.47
S$13885
  Bottom 0: 191.45,129.47 191.66,129.76
S$13886
  Bottom 0: 191.66,129.76 191.78,130.08
S$13887
  Bottom 0: 191.78,130.08 191.83,130.43
S$13888
  Bottom 0: 191.83,130.43 191.78,130.77
S$13889
  Bottom 0: 191.78,130.77 191.66,131.1
S$13890
  Bottom 0: 191.66,131.1 191.45,131.38
S$13891
  Bottom 0: 191.45,131.38 191.18,131.61
S$13892
  Bottom 0: 191.18,131.61 190.87,131.76
S$13893
  Bottom 0: 190.87,131.76 190.52,131.82
S$13894
  Bottom 0: 190.52,131.82 190.17,131.8
S$13895
  Bottom 0: 190.17,131.8 189.84,131.69
S$13896
  Bottom 0: 189.84,131.69 189.81,131.68
S$13897
  Bottom 0: 189.81,131.68 189.25,132.25
S$13898
  Bottom 0: 189.25,132.25 189.19,132.29
S$13899
  Bottom 0: 189.19,132.29 189.13,132.33
S$13900
  Bottom 0: 189.13,132.33 189.06,132.35
S$13901
  Bottom 0: 189.06,132.35 189,132.37
S$13902
  Bottom 0: 189,132.37 188.93,132.38
S$13903
  Bottom 0: 188.93,132.38 184.37,132.38
S$13904
  Bottom 0: 184.37,132.38 184.31,132.51
S$13905
  Bottom 0: 184.31,132.51 184.1,132.72
S$13906
  Bottom 0: 184.1,132.72 183.84,132.88
S$13907
  Bottom 0: 183.84,132.88 183.54,132.94
S$13908
  Bottom 0: 183.54,132.94 183.24,132.92
S$13909
  Bottom 0: 183.24,132.92 182.96,132.81
S$13910
  Bottom 0: 182.96,132.81 182.72,132.62
S$13911
  Bottom 0: 182.72,132.62 182.56,132.38
S$13912
  Bottom 0: 182.56,132.38 182.46,132.09
S$13913
  Bottom 0: 182.46,132.09 182.46,131.78
S$13914
  Bottom 0: 182.46,131.78 182.56,131.49
S$13915
  Bottom 0: 182.56,131.49 182.72,131.24
S$13916
  Bottom 0: 182.72,131.24 182.96,131.05
S$13917
  Bottom 0: 182.96,131.05 183.24,130.94
S$13918
  Bottom 0: 183.24,130.94 183.54,130.92
S$13919
  Bottom 0: 183.54,130.92 183.84,130.99
S$13920
  Bottom 0: 183.84,130.99 184.1,131.14
S$13921
  Bottom 0: 184.1,131.14 184.31,131.36
S$13922
  Bottom 0: 184.31,131.36 184.37,131.49
S$13923
  Bottom 0: 184.37,131.49 188.74,131.49
S$13924
  Bottom 0: 188.74,131.49 189.19,131.04
S$13925
  Bottom 0: 189.19,131.04 189.13,130.94
S$13926
  Bottom 0: 189.13,130.94 189.05,130.6
S$13927
  Bottom 0: 189.05,130.6 189.05,130.25
S$13928
  Bottom 0: 189.05,130.25 189.13,129.92
S$13929
  Bottom 0: 189.13,129.92 189.31,129.61
S$13930
  Bottom 0: 189.31,129.61 189.54,129.35
S$13931
  Bottom 0: 189.54,129.35 189.84,129.16
S$13932
  Bottom 0: 189.84,129.16 190.17,129.06
S$13933
  Bottom 0: 190.17,129.06 190.52,129.04
S$13934
  Bottom 0: 183.54,138.54 183.84,138.61
S$13935
  Bottom 0: 183.84,138.61 184.1,138.76
S$13936
  Bottom 0: 184.1,138.76 184.31,138.98
S$13937
  Bottom 0: 184.31,138.98 184.44,139.25
S$13938
  Bottom 0: 184.44,139.25 184.49,139.55
S$13939
  Bottom 0: 184.49,139.55 184.44,139.85
S$13940
  Bottom 0: 184.44,139.85 184.31,140.13
S$13941
  Bottom 0: 184.31,140.13 184.1,140.34
S$13942
  Bottom 0: 184.1,140.34 183.84,140.5
S$13943
  Bottom 0: 183.84,140.5 183.54,140.56
S$13944
  Bottom 0: 183.54,140.56 183.24,140.54
S$13945
  Bottom 0: 183.24,140.54 182.96,140.43
S$13946
  Bottom 0: 182.96,140.43 182.72,140.24
S$13947
  Bottom 0: 182.72,140.24 182.56,140
S$13948
  Bottom 0: 182.56,140 182.46,139.71
S$13949
  Bottom 0: 182.46,139.71 182.46,139.4
S$13950
  Bottom 0: 182.46,139.4 182.56,139.11
S$13951
  Bottom 0: 182.56,139.11 182.72,138.86
S$13952
  Bottom 0: 182.72,138.86 182.96,138.67
S$13953
  Bottom 0: 182.96,138.67 183.24,138.56
S$13954
  Bottom 0: 183.24,138.56 183.54,138.54
S$13955
  Bottom 0: 150.22,125.36 150.19,125.41
S$13956
  Bottom 0: 150.19,125.41 149.99,125.66
S$13957
  Bottom 0: 149.99,125.66 149.72,125.85
S$13958
  Bottom 0: 149.72,125.85 149.42,125.96
S$13959
  Bottom 0: 149.42,125.96 149.13,125.98
S$13960
  Bottom 0: 149.13,125.98 150.66,127.5
S$13961
  Bottom 0: 150.66,127.5 151.99,127.5
S$13962
  Bottom 0: 151.99,127.5 152.06,127.51
S$13963
  Bottom 0: 152.06,127.51 152.13,127.52
S$13964
  Bottom 0: 152.13,127.52 152.19,127.55
S$13965
  Bottom 0: 152.19,127.55 152.25,127.59
S$13966
  Bottom 0: 152.25,127.59 152.31,127.63
S$13967
  Bottom 0: 152.31,127.63 157.33,132.65
S$13968
  Bottom 0: 157.33,132.65 157.38,132.46
S$13969
  Bottom 0: 157.38,132.46 157.55,132.15
S$13970
  Bottom 0: 157.55,132.15 157.79,131.89
S$13971
  Bottom 0: 157.79,131.89 158.09,131.7
S$13972
  Bottom 0: 158.09,131.7 158.42,131.6
S$13973
  Bottom 0: 158.42,131.6 158.77,131.58
S$13974
  Bottom 0: 158.77,131.58 158.98,131.61
S$13975
  Bottom 0: 158.98,131.61 152.72,125.36
S$13976
  Bottom 0: 152.72,125.36 150.22,125.36
S$13977
  Bottom 0: 148.45,126.55 148.51,126.65
S$13978
  Bottom 0: 148.51,126.65 148.56,126.9
S$13979
  Bottom 0: 148.56,126.9 148.51,127.15
S$13980
  Bottom 0: 148.51,127.15 148.38,127.36
S$13981
  Bottom 0: 148.38,127.36 148.18,127.51
S$13982
  Bottom 0: 148.18,127.51 147.93,127.58
S$13983
  Bottom 0: 147.93,127.58 147.69,127.56
S$13984
  Bottom 0: 147.69,127.56 147.46,127.45
S$13985
  Bottom 0: 147.46,127.45 147.29,127.26
S$13986
  Bottom 0: 147.29,127.26 147.2,127.03
S$13987
  Bottom 0: 147.2,127.03 147.2,126.85
S$13988
  Bottom 0: 147.2,126.85 147.19,126.84
S$13989
  Bottom 0: 147.19,126.84 147.19,130.83
S$13990
  Bottom 0: 147.19,130.83 152.79,136.43
S$13991
  Bottom 0: 152.79,136.43 152.76,136.38
S$13992
  Bottom 0: 152.76,136.38 152.63,135.96
S$13993
  Bottom 0: 152.63,135.96 152.59,135.51
S$13994
  Bottom 0: 152.59,135.51 152.63,135.06
S$13995
  Bottom 0: 152.63,135.06 152.76,134.63
S$13996
  Bottom 0: 152.76,134.63 152.97,134.24
S$13997
  Bottom 0: 152.97,134.24 153.26,133.89
S$13998
  Bottom 0: 153.26,133.89 153.6,133.61
S$13999
  Bottom 0: 153.6,133.61 154,133.4
S$14000
  Bottom 0: 154,133.4 154.43,133.27
S$14001
  Bottom 0: 154.43,133.27 154.87,133.22
S$14002
  Bottom 0: 154.87,133.22 155.32,133.27
S$14003
  Bottom 0: 155.32,133.27 155.75,133.4
S$14004
  Bottom 0: 155.75,133.4 156.14,133.61
S$14005
  Bottom 0: 156.14,133.61 156.49,133.89
S$14006
  Bottom 0: 156.49,133.89 156.66,134.11
S$14007
  Bottom 0: 156.66,134.11 156.66,133.25
S$14008
  Bottom 0: 156.66,133.25 153.71,130.29
S$14009
  Bottom 0: 153.71,130.29 153.73,130.43
S$14010
  Bottom 0: 153.73,130.43 153.68,130.77
S$14011
  Bottom 0: 153.68,130.77 153.56,131.1
S$14012
  Bottom 0: 153.56,131.1 153.35,131.38
S$14013
  Bottom 0: 153.35,131.38 153.08,131.61
S$14014
  Bottom 0: 153.08,131.61 152.77,131.76
S$14015
  Bottom 0: 152.77,131.76 152.42,131.82
S$14016
  Bottom 0: 152.42,131.82 152.07,131.8
S$14017
  Bottom 0: 152.07,131.8 151.74,131.69
S$14018
  Bottom 0: 151.74,131.69 151.44,131.51
S$14019
  Bottom 0: 151.44,131.51 151.2,131.25
S$14020
  Bottom 0: 151.2,131.25 151.03,130.94
S$14021
  Bottom 0: 151.03,130.94 150.95,130.6
S$14022
  Bottom 0: 150.95,130.6 150.95,130.25
S$14023
  Bottom 0: 150.95,130.25 151.03,129.92
S$14024
  Bottom 0: 151.03,129.92 151.2,129.61
S$14025
  Bottom 0: 151.2,129.61 151.44,129.35
S$14026
  Bottom 0: 151.44,129.35 151.74,129.16
S$14027
  Bottom 0: 151.74,129.16 152.07,129.06
S$14028
  Bottom 0: 152.07,129.06 152.42,129.04
S$14029
  Bottom 0: 152.42,129.04 152.47,129.04
S$14030
  Bottom 0: 152.47,129.04 151.81,128.39
S$14031
  Bottom 0: 151.81,128.39 150.47,128.39
S$14032
  Bottom 0: 150.47,128.39 150.4,128.38
S$14033
  Bottom 0: 150.4,128.38 150.34,128.37
S$14034
  Bottom 0: 150.34,128.37 150.28,128.34
S$14035
  Bottom 0: 150.28,128.34 150.22,128.3
S$14036
  Bottom 0: 150.22,128.3 150.16,128.26
S$14037
  Bottom 0: 150.16,128.26 148.45,126.55
S$14038
  Bottom 0: 146.28,131.52 146.33,131.63
S$14039
  Bottom 0: 146.33,131.63 146.38,131.93
S$14040
  Bottom 0: 146.38,131.93 146.33,132.23
S$14041
  Bottom 0: 146.33,132.23 146.2,132.51
S$14042
  Bottom 0: 146.2,132.51 145.99,132.72
S$14043
  Bottom 0: 145.99,132.72 145.73,132.88
S$14044
  Bottom 0: 145.73,132.88 145.44,132.94
S$14045
  Bottom 0: 145.44,132.94 145.28,132.93
S$14046
  Bottom 0: 145.28,132.93 150.09,137.74
S$14047
  Bottom 0: 150.09,137.74 150.13,137.79
S$14048
  Bottom 0: 150.13,137.79 150.17,137.86
S$14049
  Bottom 0: 150.17,137.86 150.19,137.92
S$14050
  Bottom 0: 150.19,137.92 150.21,137.98
S$14051
  Bottom 0: 150.21,137.98 150.22,138.05
S$14052
  Bottom 0: 150.22,138.05 150.22,143.04
S$14053
  Bottom 0: 150.22,143.04 150.39,142.87
S$14054
  Bottom 0: 150.39,142.87 150.68,142.72
S$14055
  Bottom 0: 150.68,142.72 151,142.66
S$14056
  Bottom 0: 151,142.66 151.33,142.68
S$14057
  Bottom 0: 151.33,142.68 151.55,142.75
S$14058
  Bottom 0: 151.55,142.75 152.6,141.7
S$14059
  Bottom 0: 152.6,141.7 152.57,141.68
S$14060
  Bottom 0: 152.57,141.68 152.51,141.62
S$14061
  Bottom 0: 152.51,141.62 152.47,141.55
S$14062
  Bottom 0: 152.47,141.55 152.46,141.48
S$14063
  Bottom 0: 152.46,141.48 152.46,139.7
S$14064
  Bottom 0: 152.46,139.7 152.47,139.62
S$14065
  Bottom 0: 152.47,139.62 152.51,139.55
S$14066
  Bottom 0: 152.51,139.55 152.57,139.5
S$14067
  Bottom 0: 152.57,139.5 152.64,139.46
S$14068
  Bottom 0: 152.64,139.46 152.72,139.45
S$14069
  Bottom 0: 152.72,139.45 154.2,139.45
S$14070
  Bottom 0: 154.2,139.45 146.28,131.52
S$14071
  Bottom 0: 236.26,132.82 236.28,132.97
S$14072
  Bottom 0: 236.28,132.97 236.24,133.31
S$14073
  Bottom 0: 236.24,133.31 236.11,133.64
S$14074
  Bottom 0: 236.11,133.64 235.9,133.92
S$14075
  Bottom 0: 235.9,133.92 235.63,134.15
S$14076
  Bottom 0: 235.63,134.15 235.32,134.3
S$14077
  Bottom 0: 235.32,134.3 234.97,134.36
S$14078
  Bottom 0: 234.97,134.36 234.62,134.34
S$14079
  Bottom 0: 234.62,134.34 234.29,134.23
S$14080
  Bottom 0: 234.29,134.23 234,134.05
S$14081
  Bottom 0: 234,134.05 233.76,133.79
S$14082
  Bottom 0: 233.76,133.79 233.58,133.48
S$14083
  Bottom 0: 233.58,133.48 233.57,133.42
S$14084
  Bottom 0: 233.57,133.42 231.98,133.42
S$14085
  Bottom 0: 231.98,133.42 232.34,133.61
S$14086
  Bottom 0: 232.34,133.61 232.69,133.89
S$14087
  Bottom 0: 232.69,133.89 232.97,134.24
S$14088
  Bottom 0: 232.97,134.24 233.19,134.63
S$14089
  Bottom 0: 233.19,134.63 233.31,135.06
S$14090
  Bottom 0: 233.31,135.06 233.36,135.51
S$14091
  Bottom 0: 233.36,135.51 233.31,135.96
S$14092
  Bottom 0: 233.31,135.96 233.19,136.38
S$14093
  Bottom 0: 233.19,136.38 232.97,136.78
S$14094
  Bottom 0: 232.97,136.78 232.69,137.12
S$14095
  Bottom 0: 232.69,137.12 232.34,137.41
S$14096
  Bottom 0: 232.34,137.41 231.95,137.62
S$14097
  Bottom 0: 231.95,137.62 231.52,137.75
S$14098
